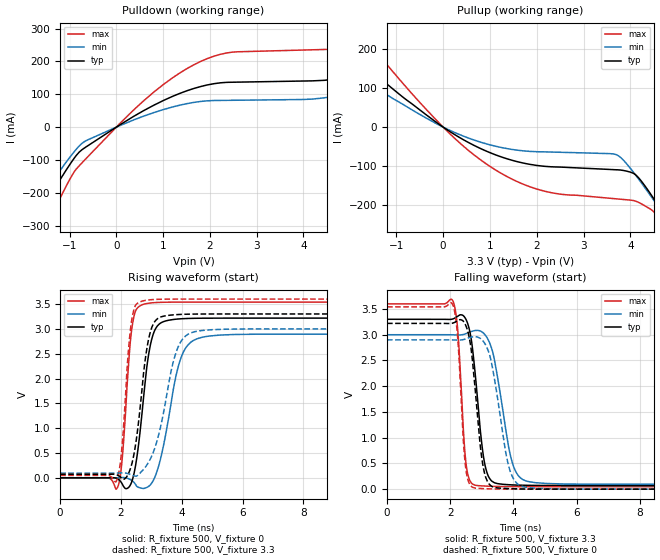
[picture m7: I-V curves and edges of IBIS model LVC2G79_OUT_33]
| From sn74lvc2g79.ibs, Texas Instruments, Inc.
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[Model]   LVC2G79_OUT_33
Model_type  Output
Vref =   0
Rref =   500
Cref =   50p
Vmeas =   1.5
| variable   typ   min   max
C_comp   9.52pF   5.86pF   13.14pF
| C_pullup   9.85pF   5.86pF   11.98pF
| C_pulldown   9.19pF   6.46pF   13.14pF
[Temperature Range]   40   100   -40
| Ambient temperature   25   85   -40
[Voltage range]   3.3   3   3.6
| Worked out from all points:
|   slope of the pulldown table from 0 to 0.495 V, typ, clamps not added: 11.5 ohm
|   slope of the pullup table from 0 to 0.495 V, typ, clamps not added: 13.6 ohm
|   rising waveform, R_fixture 500, V_fixture 0: 20-80 % time 362ps typ, 546ps min, 240ps max; typ from 0 V to 3.22 V
|   falling waveform, R_fixture 500, V_fixture 3.3: 20-80 % time 314ps typ, 470ps min, 197ps max; typ from 3.3 V to 0.071 V
|   rising waveform, R_fixture 500, V_fixture 3.3: 20-80 % time 374ps typ, 604ps min, 243ps max; typ from 0.07 V to 3.3 V
|   falling waveform, R_fixture 500, V_fixture 0: 20-80 % time 301ps typ, 452ps min, 195ps max; typ from 3.22 V to 0 V
[Pulldown]
| LVC2G79_OUT_33
|   Voltage   I(typ)   I(min)   I(max)
-5.5V     -1.107A    -970.8mA   -1.353A
-2.055V   -353.2mA   -300.4mA   -454.5mA
-1.49V    -224.6mA   -188.2mA   -296.4mA
-740mV    -69.5mA    -50.1mA    -109.7mA
365mV     32.28mA    21.63mA    51.56mA
2.22V     134.9mA    81.36mA    221.6mA
4.92V     153.7mA    101.9mA    243.5mA
6.98V     278.6mA    201.4mA    397.7mA
7.35V     308.4mA    129.2mA    438.3mA
7.84V     330.1mA    92.32mA    495.6mA
8.75V     170.7mA    93.06mA    502mA
11V       160mA      96.27mA    278.2mA
[Pullup]
| LVC2G79_OUT_33
|   Voltage   I(typ)   I(min)   I(max)
-5.5V     609.5mA    479.2mA    854.2mA
-3.49V    364.8mA    283mA      516.7mA
-2.685V   271.1mA    208.6mA    386.5mA
-1.96V    190.3mA    144.9mA    273.3mA
-55mV     4.572mA    3.33mA     6.783mA
1.095V    -70.05mA   -48.34mA   -108.1mA
2.155V    -100.5mA   -63.45mA   -164.1mA
3.69V     -109.4mA   -70.27mA   -184mA
4.135V    -124.9mA   -126.7mA   -191mA
4.79V     -237.5mA   -238.3mA   -272mA
5V        -277.7mA   -275.7mA   -316.9mA
11V       -1.518A    -1.406A    -1.753A
[Ramp]
| LVC2G79_OUT_33
| variable   typ   min   max
dV/dt_r   2.06/3.90E-10   1.87/5.90E-10   2.26/2.64E-10
dV/dt_f   1.99/3.31E-10   1.79/4.93E-10   2.19/2.09E-10
R_load = 500
[Rising Waveform]
| LVC2G79_OUT_33
R_fixture =   500
C_fixture =   0
L_fixture =   0
V_fixture =   0
V_fixture_min = 0
V_fixture_max = 0
|   Time   V(typ)   V(min)   V(max)
0s        144.1pV    5.487nV    2.182nV
1.89ns    -21.15mV   1.823mV    -187.1mV
2.04ns    -121.9mV   5.94mV     383.9mV
2.365ns   -61.01mV   -57.19mV   3.041V
2.785ns   1.869V     -209.4mV   3.502V
2.975ns   2.698V     -134mV     3.522V
3.205ns   3.065V     168.4mV    3.532V
3.945ns   3.201V     2.366V     3.538V
4.63ns    3.214V     2.825V     3.539V
22.5ns    3.216V     2.894V     3.539V
[Falling Waveform]
| LVC2G79_OUT_33
R_fixture =   500
C_fixture =   0
L_fixture =   0
V_fixture =   3.3
V_fixture_min = 3
V_fixture_max = 3.6
|   Time   V(typ)   V(min)   V(max)
0s        3.3V       3V         3.6V
2.09ns    3.308V     2.998V     3.651V
2.24ns    3.361V     2.995V     3.072V
2.5ns     3.295V     3.022V     497.9mV
2.79ns    2.242V     3.081V     76.83mV
3.02ns    775.6mV    3.048V     63.27mV
3.205ns   252.2mV    2.897V     57.48mV
3.955ns   83.27mV    535.7mV    49.6mV
4.47ns    74.51mV    147.6mV    48.78mV
22.5ns    70.51mV    94.58mV    48.43mV
[Rising Waveform]
| LVC2G79_OUT_33
R_fixture =   500
C_fixture =   0
L_fixture =   0
V_fixture =   3.3
V_fixture_min = 3
V_fixture_max = 3.6
|   Time   V(typ)   V(min)   V(max)
0s        70.47mV    94.51mV    48.4mV
1.85ns    63.28mV    95.69mV    -67.37mV
2.02ns    -4.211mV   100.3mV    537.1mV
2.345ns   254.9mV    58mV       3.146V
2.715ns   1.93V      152.4mV    3.561V
2.9ns     2.768V     307mV      3.582V
3.115ns   3.151V     602mV      3.592V
3.81ns    3.286V     2.523V     3.599V
4.42ns    3.298V     2.942V     3.6V
22.5ns    3.3V       3V         3.6V
[Falling Waveform]
| LVC2G79_OUT_33
R_fixture =   500
C_fixture =   0
L_fixture =   0
V_fixture =   0
V_fixture_min = 0
V_fixture_max = 0
|   Time   V(typ)   V(min)   V(max)
0s        3.22V      2.9V       3.542V
2.08ns    3.226V     2.898V     3.583V
2.23ns    3.271V     2.896V     2.989V
2.485ns   3.189V     2.918V     435.2mV
2.78ns    2.001V     2.961V     21.8mV
2.985ns   665.6mV    2.913V     12.16mV
3.175ns   152.4mV    2.731V     7.647mV
3.85ns    10.94mV    447.4mV    1.242mV
4.32ns    3.638mV    46.19mV    431.1uV
22.5ns    39.69uV    54.54uV    27.91uV
